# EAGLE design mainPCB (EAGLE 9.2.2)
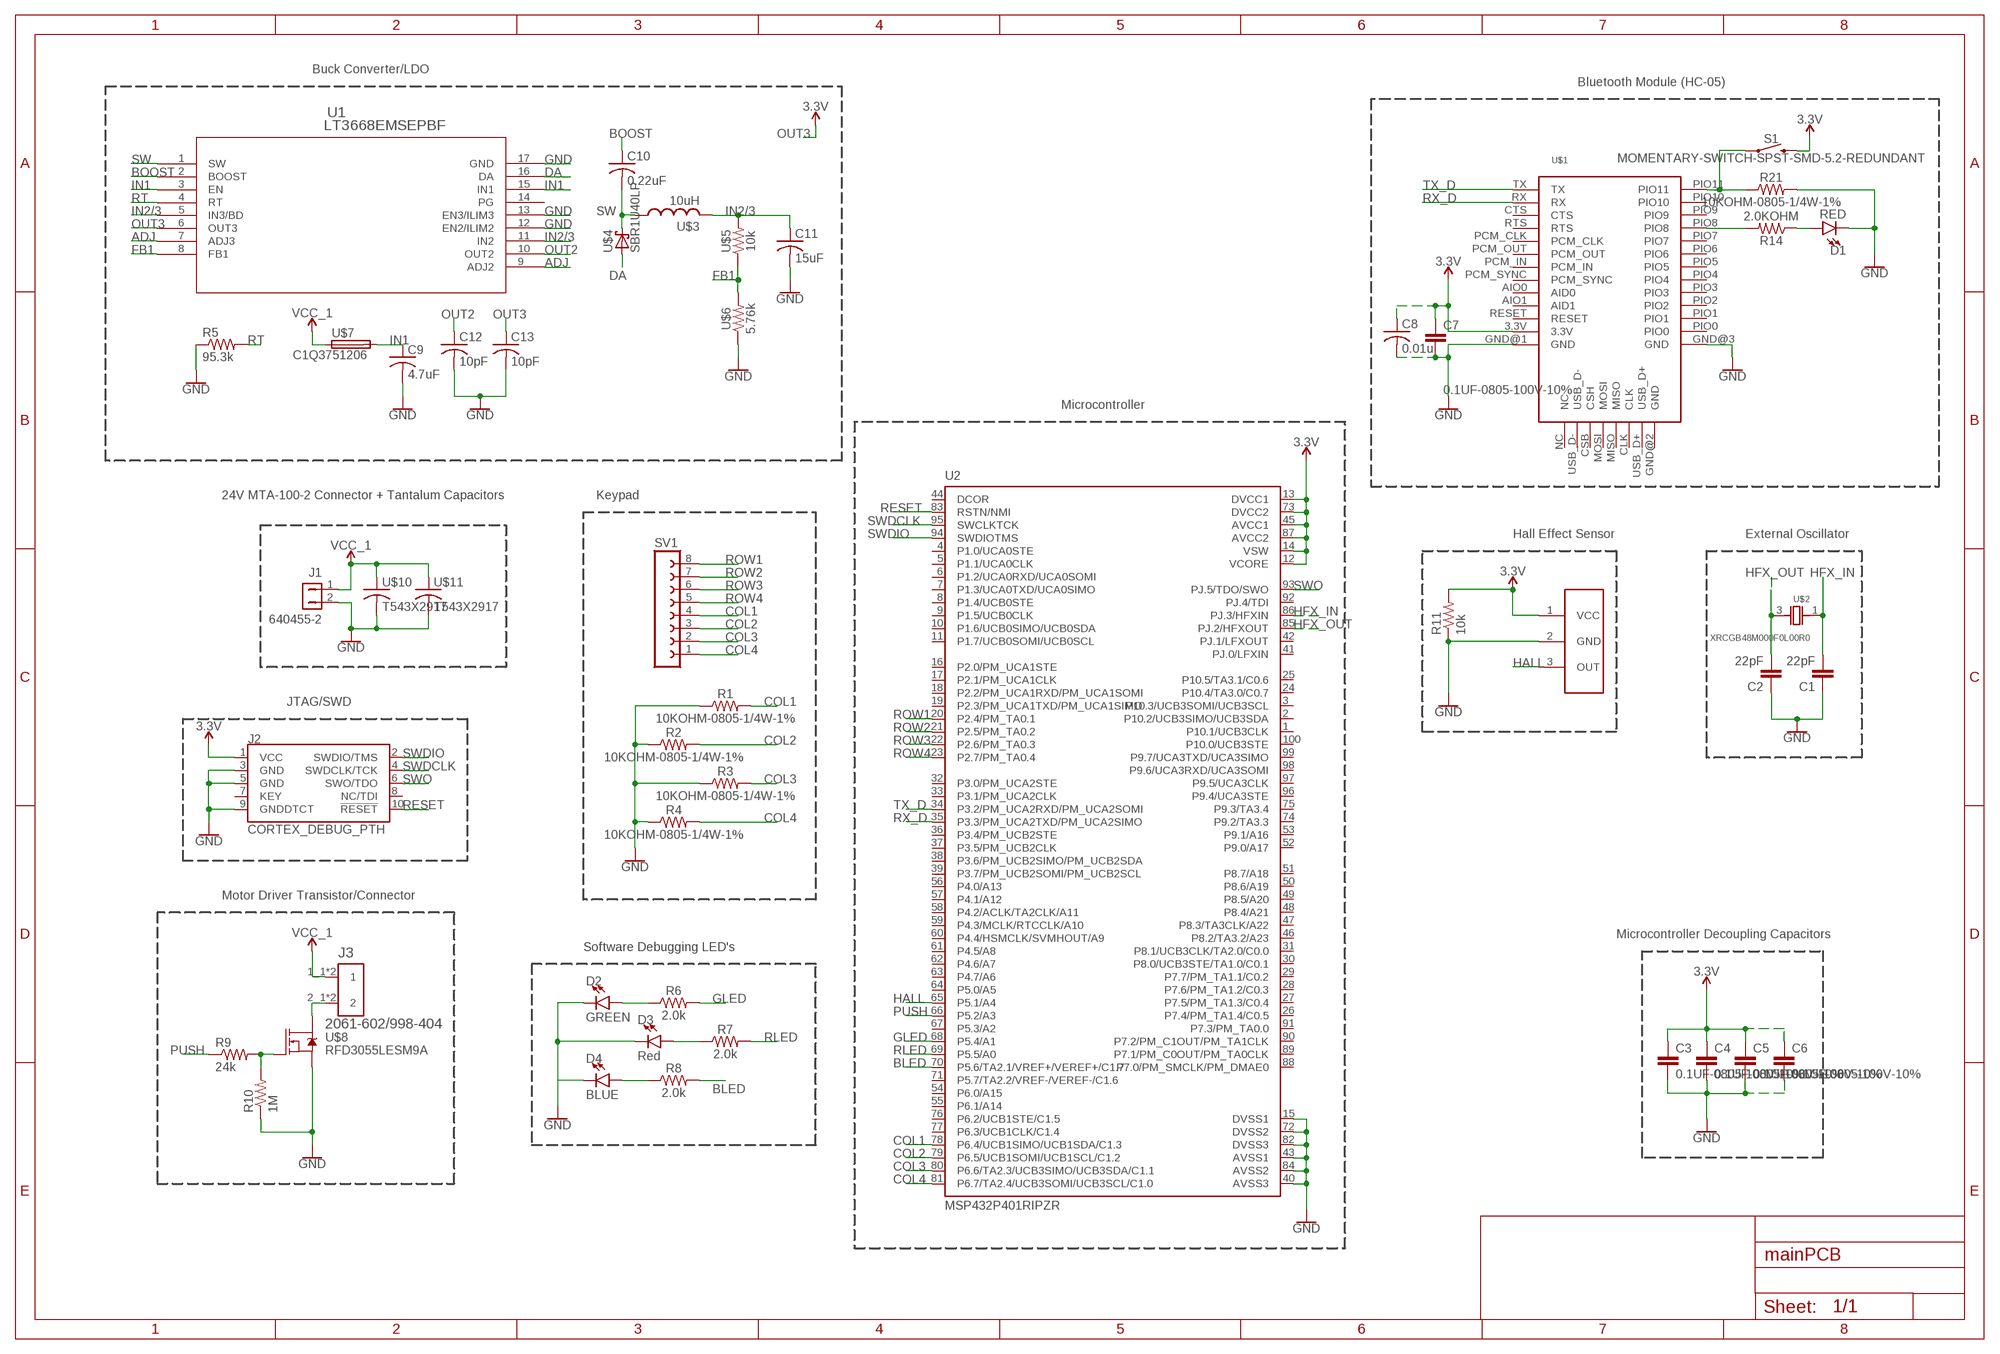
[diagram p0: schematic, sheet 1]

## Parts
C1  22pF  22PF-0603-50V-5%  [0603]
C2  22pF  22PF-0603-50V-5%  [0603]
C3  0.1UF-0805-100V-10%  [0805]
C4  0.1UF-0805-100V-10%  [0805]
C5  0.1UF-0805-100V-10%  [0805]
C6  0.1UF-0805-100V-10%  [0805]
C7  0.1UF-0805-100V-10%  [0805]
C8  0.01u  C-USC0805  [C0805]
C9  4.7uF  C-USC0805  [C0805]
C10  0.22uF  C-USC0805  [C0805]
C11  15uF  C-USC0805  [C0805]
C12  10pF  C-USC0805  [C0805]
C13  10pF  C-USC0805  [C0805]
D1  RED  LED-RED0603  [LED-0603]
D2  GREEN  LED-GREEN0603  [LED-0603]
D3  Red  LED-RED0603-SMART  [LED-0603]
D4  BLUE  LED-BLUE0603  [LED-0603]
J1  640455-2  [2-PIN_CONNECTOR]
J2  CORTEX_DEBUG_PTH  [2X5-PTH-1.27MM]
J3  2061-602/998-404  [WAGO_2061-602/998-404]
R1  10KOHM-0805-1/4W-1%  [0805]
R2  10KOHM-0805-1/4W-1%  [0805]
R3  10KOHM-0805-1/4W-1%  [0805]
R4  10KOHM-0805-1/4W-1%  [0805]
R5  95.3k  R-US_R0805  [R0805]
R6  2.0k  2.0KOHM-0603-1/10W-5%  [0603]
R7  2.0k  2.0KOHM-0603-1/10W-5%  [0603]
R8  2.0k  2.0KOHM-0603-1/10W-5%  [0603]
R9  24k  R-US_R0805  [R0805]
R10  1M  R-US_R0805  [R0805]
R11  10k  R-US_R0805  [R0805]
R14  2.0KOHM  [0805]
R21  10KOHM-0805-1/4W-1%  [0805]
S1  MOMENTARY-SWITCH-SPST-SMD-5.2-REDUNDANT  [TACTILE_SWITCH_SMD_5.2MM]
SV1  FE08-1  [FE08]
U1  LT3668EMSEPBF  [MSOP-16_MSE]
U2  MSP432P401RIPZR  [QFP50P1600X1600X160-100N]
U$1  HC-05  [HC-05_FOOTPRINT]
U$2  XRCGB48M000F0L00R0  [XTAL_XRCGB24M000F0L00R0]
U$3  10uH  CBC3225T150KR1210  [L3225M]
U$4  SBR1U40LP  [3-XDFN]
U$5  10k  ERJ-PB6  [R0805]
U$6  5.76k  ERJ-PB6  [R0805]
U$7  C1Q3751206  [C1206]
U$8  RFD3055LESM9A  [DPAK229P990X239-4N]
U$9  AH1807-P-B  [SIP3-UA]
U$10  T543X2917  [0204/5]
U$11  T543X2917  [0204/5]

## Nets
3.3V: C3.1 C4.1 C5.1 C6.1 C7.1 C8.1 J2.1(VCC) R11.2 S1.3 S1.4 U2.12(VCORE) U2.13(DVCC1) U2.14(VSW) U2.45(AVCC1) U2.73(DVCC2) U2.87(AVCC2) U$1.3.3V U$9.1(VCC)
ADJ: U1.7(ADJ3) U1.9(ADJ2)
BLED: R8.2 U2.70(P5.6/TA2.1/VREF+/VEREF+/C1.7)
BOOST: C10.1 U1.2(BOOST)
COL1: R1.2 SV1.4 U2.78(P6.4/UCB1SIMO/UCB1SDA/C1.3)
COL2: R2.2 SV1.3 U2.79(P6.5/UCB1SOMI/UCB1SCL/C1.2)
COL3: R3.2 SV1.2 U2.80(P6.6/TA2.3/UCB3SIMO/UCB3SDA/C1.1)
COL4: R4.2 SV1.1 U2.81(P6.7/TA2.4/UCB3SOMI/UCB3SCL/C1.0)
DA: U1.16(DA) U$4.1(A)
FB1: U1.8(FB1) U$5.1 U$6.2
GLED: R6.2 U2.68(P5.4/A1)
GND: C1.1 C2.1 C3.2 C4.2 C5.2 C6.2 C7.2 C8.2 C9.2 C11.2 C12.2 C13.2 D1.C D2.C D3.C J1.2 J2.3(GND) J2.5(GND) J2.9(GNDDTCT) R1.1 R2.1 R3.1 R4.1 R5.1 R10.1 R11.1 R21.2 U1.12(EN2/ILIM2) U1.13(EN3/ILIM3) U1.17(GND) U2.15(DVSS1) U2.40(AVSS3) U2.43(AVSS1) U2.72(DVSS2) U2.82(DVSS3) U2.84(AVSS2) U$1.GND@1(GND) U$1.GND@3(GND) U$6.1 U$8.3(S) U$9.2(GND) U$10.2 U$11.2
HALL: U2.65(P5.1/A4) U$9.3(OUT)
HFX_IN: C1.2 U2.86(PJ.3/HFXIN) U$2.1
HFX_OUT: C2.2 U2.85(PJ.2/HFXOUT) U$2.3
IN1: C9.1 U1.3(EN) U1.15(IN1) U$7.2
IN2/3: C11.1 U1.5(IN3/BD) U1.11(IN2) U$3.2 U$5.2
N$1: R9.2 R10.2 U$8.1(G)
N$2: J3.2_1 J3.2_2 U$8.4(D)
N$3: D1.A R14.1
N$4: D2.A R6.1
N$5: D3.A R7.1
N$8: D4.A R8.1
N$9: D4.C
N$11: R21.1 S1.1 S1.2 U$1.PIO11
N$19: R14.2 U$1.PIO8
OUT2: C12.1 U1.10(OUT2)
OUT3: C13.1 U1.6(OUT3) ; supply symbol labelled 3.3V
PUSH: R9.1 U2.66(P5.2/A3)
RESET: J2.10(!RESET) U2.83(RSTN/NMI)
RLED: R7.2 U2.69(P5.5/A0)
ROW1: SV1.8 U2.20(P2.4/PM_TA0.1)
ROW2: SV1.7 U2.21(P2.5/PM_TA0.2)
ROW3: SV1.6 U2.22(P2.6/PM_TA0.3)
ROW4: SV1.5 U2.23(P2.7/PM_TA0.4)
RT: R5.2 U1.4(RT)
RX_D: U2.35(P3.3/PM_UCA2TXD/PM_UCA2SIMO) U$1.RX
SW: C10.2 U1.1(SW) U$3.1 U$4.2(C) U$4.3(C)
SWDCLK: J2.4(SWDCLK/TCK) U2.95(SWCLKTCK)
SWDIO: J2.2(SWDIO/TMS) U2.94(SWDIOTMS)
SWO: J2.6(SWO/TDO) U2.93(PJ.5/TDO/SWO)
TX_D: U2.34(P3.2/PM_UCA2RXD/PM_UCA2SOMI) U$1.TX
VCC_1: J1.1 J3.1_1 J3.1_2 U$7.1 U$10.1 U$11.1
Unconnected: J2.7(KEY) J2.8(NC/TDI) U1.14(PG) U2.1(P10.1/UCB3CLK) U2.2(P10.2/UCB3SIMO/UCB3SDA) U2.3(P10.3/UCB3SOMI/UCB3SCL) U2.4(P1.0/UCA0STE) U2.5(P1.1/UCA0CLK) U2.6(P1.2/UCA0RXD/UCA0SOMI) U2.7(P1.3/UCA0TXD/UCA0SIMO) U2.8(P1.4/UCB0STE) U2.9(P1.5/UCB0CLK) U2.10(P1.6/UCB0SIMO/UCB0SDA) U2.11(P1.7/UCB0SOMI/UCB0SCL) U2.16(P2.0/PM_UCA1STE) U2.17(P2.1/PM_UCA1CLK) U2.18(P2.2/PM_UCA1RXD/PM_UCA1SOMI) U2.19(P2.3/PM_UCA1TXD/PM_UCA1SIMO) U2.24(P10.4/TA3.0/C0.7) U2.25(P10.5/TA3.1/C0.6) U2.26(P7.4/PM_TA1.4/C0.5) U2.27(P7.5/PM_TA1.3/C0.4) U2.28(P7.6/PM_TA1.2/C0.3) U2.29(P7.7/PM_TA1.1/C0.2) U2.30(P8.0/UCB3STE/TA1.0/C0.1) U2.31(P8.1/UCB3CLK/TA2.0/C0.0) U2.32(P3.0/PM_UCA2STE) U2.33(P3.1/PM_UCA2CLK) U2.36(P3.4/PM_UCB2STE) U2.37(P3.5/PM_UCB2CLK) U2.38(P3.6/PM_UCB2SIMO/PM_UCB2SDA) U2.39(P3.7/PM_UCB2SOMI/PM_UCB2SCL) U2.41(PJ.0/LFXIN) U2.42(PJ.1/LFXOUT) U2.44(DCOR) U2.46(P8.2/TA3.2/A23) U2.47(P8.3/TA3CLK/A22) U2.48(P8.4/A21) U2.49(P8.5/A20) U2.50(P8.6/A19) U2.51(P8.7/A18) U2.52(P9.0/A17) U2.53(P9.1/A16) U2.54(P6.0/A15) U2.55(P6.1/A14) U2.56(P4.0/A13) U2.57(P4.1/A12) U2.58(P4.2/ACLK/TA2CLK/A11) U2.59(P4.3/MCLK/RTCCLK/A10) U2.60(P4.4/HSMCLK/SVMHOUT/A9) U2.61(P4.5/A8) U2.62(P4.6/A7) U2.63(P4.7/A6) U2.64(P5.0/A5) U2.67(P5.3/A2) U2.71(P5.7/TA2.2/VREF-/VEREF-/C1.6) U2.74(P9.2/TA3.3) U2.75(P9.3/TA3.4) U2.76(P6.2/UCB1STE/C1.5) U2.77(P6.3/UCB1CLK/C1.4) U2.88(P7.0/PM_SMCLK/PM_DMAE0) U2.89(P7.1/PM_C0OUT/PM_TA0CLK) U2.90(P7.2/PM_C1OUT/PM_TA1CLK) U2.91(P7.3/PM_TA0.0) U2.92(PJ.4/TDI) U2.96(P9.4/UCA3STE) U2.97(P9.5/UCA3CLK) U2.98(P9.6/UCA3RXD/UCA3SOMI) U2.99(P9.7/UCA3TXD/UCA3SIMO) U2.100(P10.0/UCB3STE) U$1.AIO0(AID0) U$1.AIO1(AID1) U$1.CLK U$1.CSB(CSH) U$1.CTS U$1.GND@2(GND) U$1.MISO U$1.MOSI U$1.NC U$1.PCM_CLK U$1.PCM_IN U$1.PCM_OUT U$1.PCM_SYNC U$1.PIO0 U$1.PIO1 U$1.PIO2 U$1.PIO3 U$1.PIO4 U$1.PIO5 U$1.PIO6 U$1.PIO7 U$1.PIO9 U$1.PIO10 U$1.RESET U$1.RTS U$1.USB_D+ U$1.USB_D-

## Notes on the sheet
- Buck Converter/LDO
- Bluetooth Module (HC-05)
- Microcontroller
- 24V MTA-100-2 Connector + Tantalum Capacitors | Keypad
- Hall Effect Sensor | External Oscillator
- JTAG/SWD
- Motor Driver Transistor/Connector
- Microcontroller Decoupling Capacitors
- Software Debugging LED's

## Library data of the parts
C1 C2 = SparkFun-Capacitors:22PF: 22pF ceramic capacitors; PROD_ID: CAP-07876
C3-C7 = SENIOR_DESIGN_COMPONENTS:0.1UF: 0.1µF ceramic capacitors
C8-C13 = SENIOR_DESIGN_COMPONENTS:C-US: CAPACITOR, American symbol; SPICEPREFIX: C
D1 = SENIOR_DESIGN_COMPONENTS:LED-RED: Red SMD LED; PROD_ID: DIO-00819
D2 = SENIOR_DESIGN_COMPONENTS:LED-GREEN: Green SMD LED; PROD_ID: DIO-00821
D3 = SENIOR_DESIGN_COMPONENTS:LED-RED: Red SMD LED; PROD_ID: DIO-11154
D4 = SENIOR_DESIGN_COMPONENTS:LED-BLUE: Blue SMD LED; PROD_ID: DIO-08575
J1 = SENIOR_DESIGN_COMPONENTS:640455-2: 2 Pin Rectangular Connector; AVAILABILITY: Unavailable; COMMENT: 640455-2; DESCRIPTION: MTA-100 2 Position 2.54 mm Single Row Right Angle Wire to Board Header; EU_ROHS_COMPLIANCE: Compliant; MF: TE Connectivity; MP: 640455-2; PACKAGE: None; PRICE: None; TE_PURCHASE_URL: https://www.te.com/usa-en/product-640455-2.html?te_bu=Cor&te_type=disp&te_campaign=seda_glo_cor-seda-global-disp-prtnr-fy19-seda-model-bom-cta_sma-317_1&elqCampaignId=32493
J2 = SparkFun-Connectors:CORTEX_DEBUG: Cortex Debug Connector - 10 pin Supports JTAG debug, Serial Wire debug, and Serial Wire Viewer. PTH and SMD connector options available. General Connector Information Products: PTH Connector -via Digi-Key SparkFun PSoc SparkFun T
J3 = SENIOR_DESIGN_COMPONENTS:2061-602/998-404: 2061 Series 2 Position 20-16 AWG 6 mm Spacing Surface Mount Terminal Block; AVAILABILITY: Unavailable; DESCRIPTION: 2061 Series 2 Position 20-16 AWG 6 mm Spacing Surface Mount Terminal Block; MF: WAGO; MP: 2061-602/998-404; PACKAGE: None; PRICE: None
R1-R4 R21 = SENIOR_DESIGN_COMPONENTS:10KOHM: 10kΩ resistor
R5 R9-R11 = SENIOR_DESIGN_COMPONENTS:R-US_: RESISTOR, American symbol; SPICEPREFIX: R
R6-R8 = SENIOR_DESIGN_COMPONENTS:2.0KOHM: 2kΩ resistor; PROD_ID: RES-08296
R14 = SENIOR_DESIGN_COMPONENTS:2.0KOHM: 2kΩ resistor
S1 = SENIOR_DESIGN_COMPONENTS:MOMENTARY-SWITCH-SPST: Momentary Switch (Pushbutton) - SPST; PROD_ID: SWCH-08247; SF_SKU: COM-08720
SV1 = SENIOR_DESIGN_COMPONENTS:FE08-1: FEMALE HEADER; OC_FARNELL: unknown; OC_NEWARK: unknown
U1 = SENIOR_DESIGN_COMPONENTS:LT3668EMSEPBF; DESCRIPTION: LT3668 - 40V 400mA Step-Down Switching Regulator with Dual Fault Protected Tracking LDOs; DIGI-KEY_PART_NUMBER: LT3668EMSE#PBF-ND; DIGI-KEY_PURCHASE_URL: https://www.digikey.com/product-detail/en/linear-technology-analog-devices/LT3668EMSE-PBF/LT3668EMSE-PBF-ND/5030729?utm_source=snapeda&utm_medium=aggregator&utm_campaign=symbol; MF: Linear Technology; MP: LT3668EMSE#PBF; PACKAGE: MSOP-16 Linear Technology
U2 = SENIOR_DESIGN_COMPONENTS:MSP432P401RIPZR: Low-Power and High Performance 32-Bit ARM Cortex M4F With 256KB Flash and 64KB RAM 100-LQFP -40 to 85; AVAILABILITY: Unavailable; DESCRIPTION: Low-Power and High Performance 32-Bit ARM Cortex M4F With 256KB Flash and 64KB RAM 100-LQFP -40 to 85; MF: Texas Instruments; MP: MSP432P401RIPZR; PACKAGE: LQFP-100 Texas Instruments; PRICE: None
U$1 = SENIOR_DESIGN_COMPONENTS:HC-05
U$2 = SENIOR_DESIGN_COMPONENTS:XRCGB48M000F0L00R0
U$3 = SENIOR_DESIGN_COMPONENTS:CBC3225T150KR
U$4 = SENIOR_DESIGN_COMPONENTS:SBR1U40LP
U$5 U$6 = SENIOR_DESIGN_COMPONENTS:ERJ-PB6
U$7 = SENIOR_DESIGN_COMPONENTS:C1Q375
U$8 = SENIOR_DESIGN_COMPONENTS:RFD3055LESM9A
U$9 = SENIOR_DESIGN_COMPONENTS:AH1807-P-B
U$10 U$11 = SENIOR_DESIGN_COMPONENTS:T543X

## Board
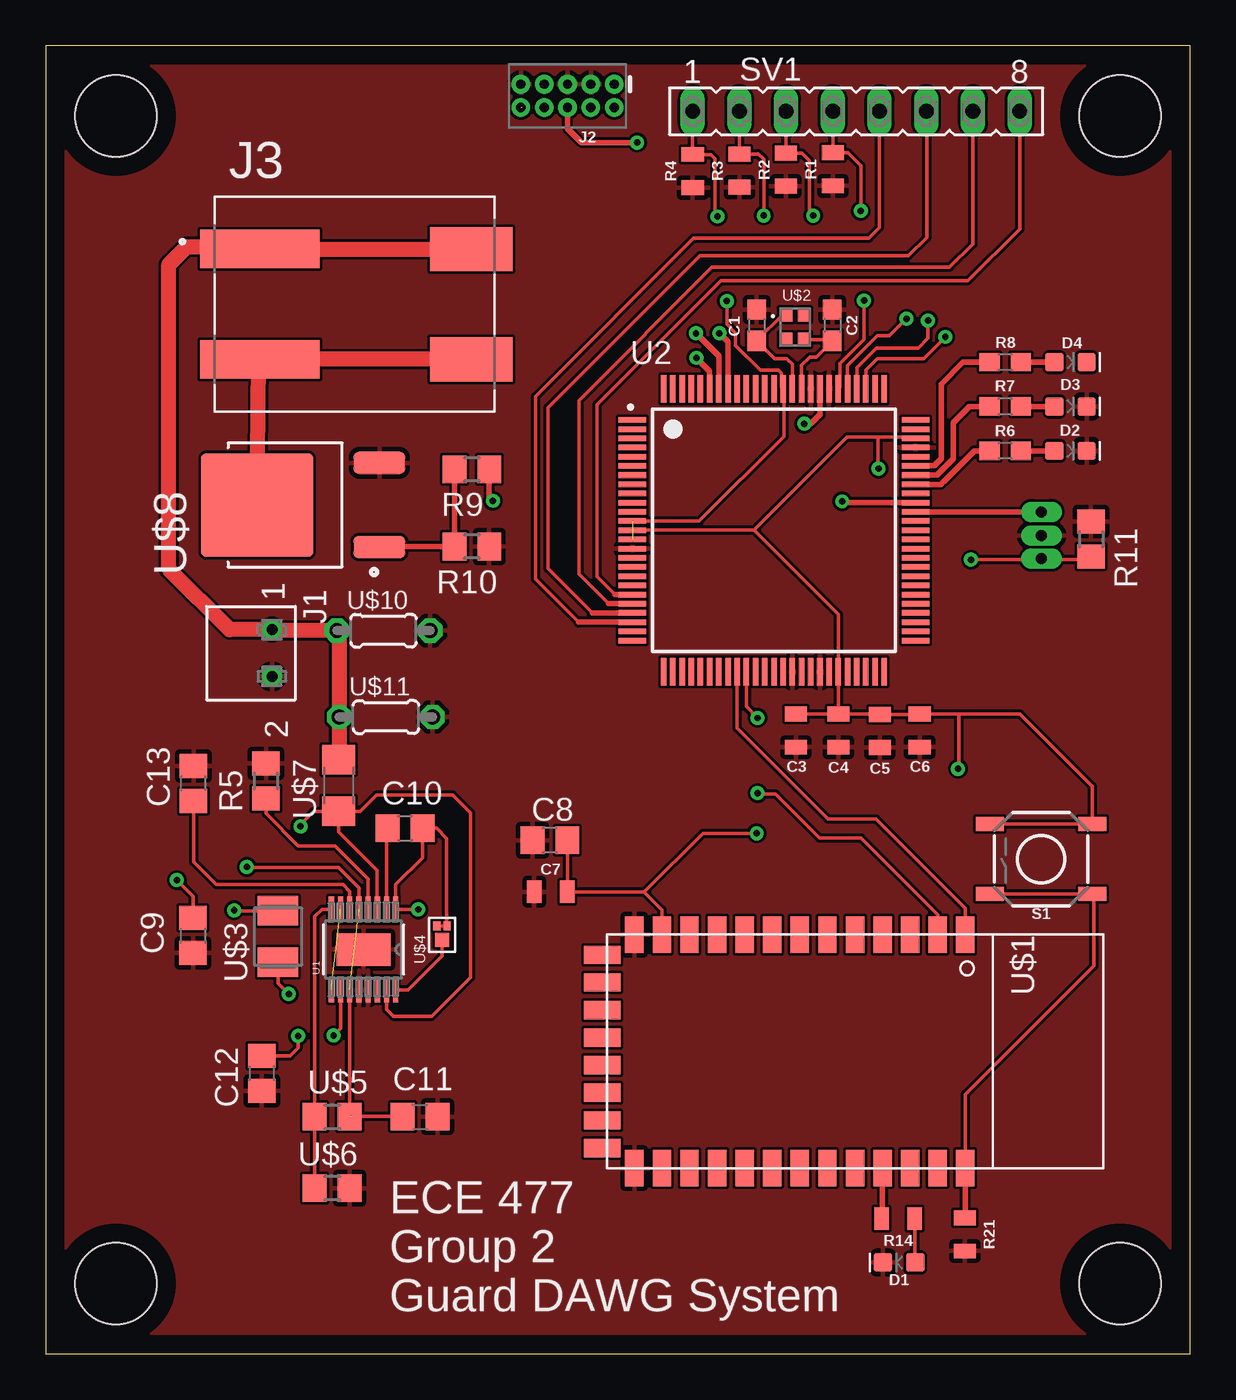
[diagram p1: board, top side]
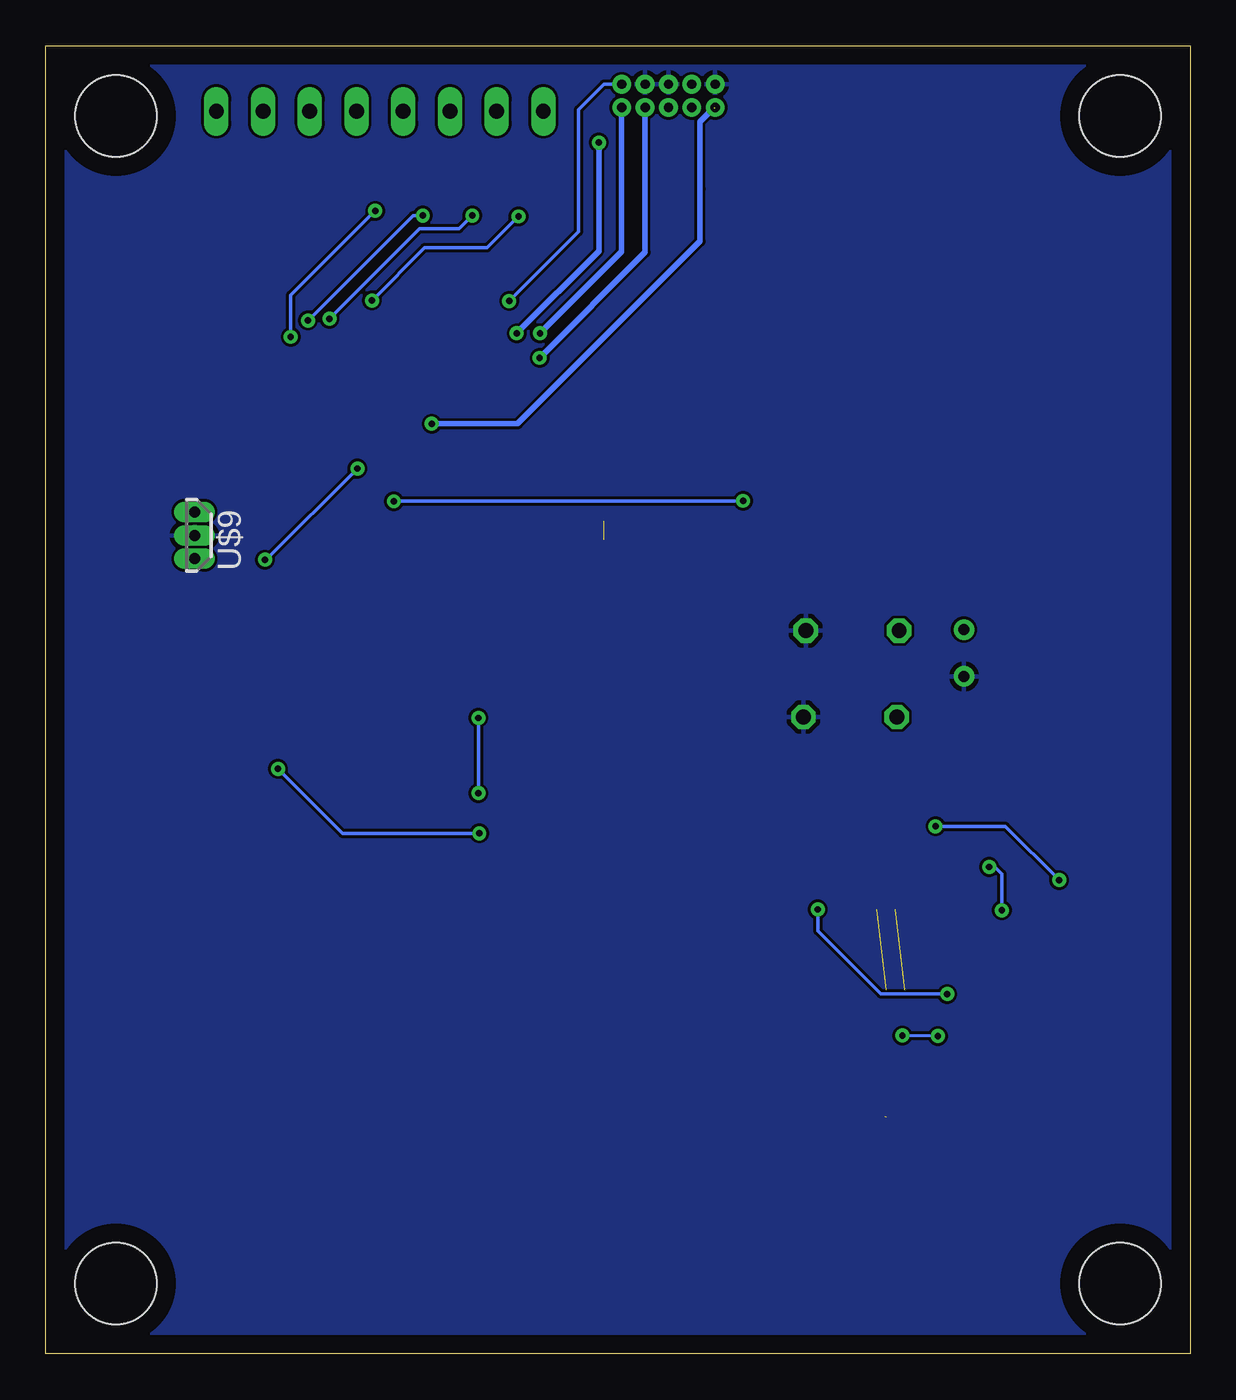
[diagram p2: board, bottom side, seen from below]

Size 62.23 x 71.12 mm. Coordinates in mm from the lower left corner, seen from the top.
Outline: 0,0 62.23,0 62.23,71.12 0,71.12 0,0
Copper layers (1*16): Top 0.035mm / dielectric 1.5mm / Bottom 0.035mm
Design rules "default": minimum track width 6mil, minimum drill 0.35mm, track to track 6mil, track to pad 6mil, pad to pad 6mil, via to via 6mil, smd to smd 6mil, copper to edge 40mil, drill to drill 6mil, minimum pad ring 10mil, minimum via ring 8mil, stop-mask expansion 4mil, vias tented up to drill 0mil, thermal gap 10mil
Holes 4.45 mm at 3.81,67.31 58.42,67.31 58.42,3.81 3.81,3.81

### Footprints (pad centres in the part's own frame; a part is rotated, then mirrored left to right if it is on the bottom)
0603 = smd 1.1 x 1: 1 -0.85,0; 2 0.85,0
0805 = smd 0.8 x 1.2: 1 -0.9,0; 2 0.9,0
C0805 = smd 1.3 x 1.5: 1 -0.95,0; 2 0.95,0
LED-0603 = smd 1 x 1: A -0.877,0; C 0.877,0
2-PIN_CONNECTOR = drill 0.6: 1 -1.27,0; 2 1.27,0
2X5-PTH-1.27MM = drill 0.508 pad 1: 1 -2.54,-0.635; 2 -2.54,0.635; 3 -1.27,-0.635; 4 -1.27,0.635; 5 0,-0.635; 6 0,0.635; 7 1.27,-0.635; 8 1.27,0.635; 9 2.54,-0.635; 10 2.54,0.635
WAGO_2061-602/998-404 = smd 6.5 x 2.1: 1_1 -5.15,3; 2_1 -5.15,-3 | smd 4.5 x 2.4: 1_2 6.35,3; 2_2 6.35,-3
R0805 = smd 1.3 x 1.5: 1 -0.95,0; 2 0.95,0
TACTILE_SWITCH_SMD_5.2MM = smd 1.524 x 0.762: 1 -2.794,1.905; 2 2.794,1.905; 3 -2.794,-1.905; 4 2.794,-1.905
FE08 = drill 0.813 long: 1 -8.89,0; 2 -6.35,0; 3 -3.81,0; 4 -1.27,0; 5 1.27,0; 6 3.81,0; 7 6.35,0; 8 8.89,0
MSOP-16_MSE = smd 1.397 x 0.279: 1 -2.184,1.751; 2 -2.184,1.251; 3 -2.184,0.751; 4 -2.184,0.25; 5 -2.184,-0.25; 6 -2.184,-0.751; 7 -2.184,-1.251; 8 -2.184,-1.751; 9 2.184,-1.751; 10 2.184,-1.251; 11 2.184,-0.751; 12 2.184,-0.25; 13 2.184,0.25; 14 2.184,0.751; 15 2.184,1.251; 16 2.184,1.751 | smd 1.753 x 2.946: 17 0,0
QFP50P1600X1600X160-100N = smd 1.5 x 0.3: 1 -7.7,6; 2 -7.7,5.5; 3 -7.7,5; 4 -7.7,4.5; 5 -7.7,4; 6 -7.7,3.5; 7 -7.7,3; 8 -7.7,2.5; 9 -7.7,2; 10 -7.7,1.5; 11 -7.7,1; 12 -7.7,0.5; 13 -7.7,0; 14 -7.7,-0.5; 15 -7.7,-1; 16 -7.7,-1.5; 17 -7.7,-2; 18 -7.7,-2.5; 19 -7.7,-3; 20 -7.7,-3.5; 21 -7.7,-4; 22 -7.7,-4.5; 23 -7.7,-5; 24 -7.7,-5.5; 25 -7.7,-6; 51 7.7,-6; 52 7.7,-5.5; 53 7.7,-5; 54 7.7,-4.5; 55 7.7,-4; 56 7.7,-3.5; 57 7.7,-3; 58 7.7,-2.5; 59 7.7,-2; 60 7.7,-1.5; 61 7.7,-1; 62 7.7,-0.5; 63 7.7,0; 64 7.7,0.5; 65 7.7,1; 66 7.7,1.5; 67 7.7,2; 68 7.7,2.5; 69 7.7,3; 70 7.7,3.5; 71 7.7,4; 72 7.7,4.5; 73 7.7,5; 74 7.7,5.5; 75 7.7,6 | smd 0.3 x 1.5: 26 -6,-7.7; 27 -5.5,-7.7; 28 -5,-7.7; 29 -4.5,-7.7; 30 -4,-7.7; 31 -3.5,-7.7; 32 -3,-7.7; 33 -2.5,-7.7; 34 -2,-7.7; 35 -1.5,-7.7; 36 -1,-7.7; 37 -0.5,-7.7; 38 0,-7.7; 39 0.5,-7.7; 40 1,-7.7; 41 1.5,-7.7; 42 2,-7.7; 43 2.5,-7.7; 44 3,-7.7; 45 3.5,-7.7; 46 4,-7.7; 47 4.5,-7.7; 48 5,-7.7; 49 5.5,-7.7; 50 6,-7.7; 76 6,7.7; 77 5.5,7.7; 78 5,7.7; 79 4.5,7.7; 80 4,7.7; 81 3.5,7.7; 82 3,7.7; 83 2.5,7.7; 84 2,7.7; 85 1.5,7.7; 86 1,7.7; 87 0.5,7.7; 88 0,7.7; 89 -0.5,7.7; 90 -1,7.7; 91 -1.5,7.7; 92 -2,7.7; 93 -2.5,7.7; 94 -3,7.7; 95 -3.5,7.7; 96 -4,7.7; 97 -4.5,7.7; 98 -5,7.7; 99 -5.5,7.7; 100 -6,7.7
HC-05_FOOTPRINT = smd 2 x 1: 3.3V 0,3; AIO0 0,7.5; AIO1 0,6; CTS 0,16.5; GND@1 0,1.5; GND@3 12.7,1.5; PCM_CLK 0,13.5; PCM_IN 0,10.5; PCM_OUT 0,12; PCM_SYNC 0,9; PIO0 12.7,3; PIO1 12.7,4.5; PIO2 12.7,6; PIO3 12.7,7.5; PIO4 12.7,9; PIO5 12.7,10.5; PIO6 12.7,12; PIO7 12.7,13.5; PIO8 12.7,15; PIO9 12.7,16.5; PIO10 12.7,18; PIO11 12.7,19.5; RESET 0,4.5; RTS 0,15; RX 0,18; TX 0,19.5 | smd 1 x 2: CLK 8.6,-0.25; CSB 4.1,-0.25; GND@2 11.6,-0.25; MISO 7.1,-0.25; MOSI 5.6,-0.25; NC 1.1,-0.25; USB_D+ 10.1,-0.25; USB_D- 2.6,-0.25
XTAL_XRCGB24M000F0L00R0 = smd 0.7 x 0.75: 1 -0.5,0.675; 2 -0.5,-0.675; 3 0.5,-0.675; 4 0.5,0.675
L3225M = smd 1.6 x 2.2: 1 -1.4,0; 2 1.4,0
3-XDFN = smd 0.75 x 0.75: 1 0,0 | smd 0.48 x 0.4: 2 0.76,0.275; 3 0.76,-0.275
C1206 = smd 1.6 x 1.8: 1 -1.4,0; 2 1.4,0
DPAK229P990X239-4N = smd 1.22 x 2.83: 1 -2.29,-4.14; 3 2.29,-4.14 | smd 5.63 x 6.1: 4 0,2.51
SIP3-UA = drill 0.6 pad 0.7 long: 1 -1.27,0; 2 0,0; 3 1.27,0
0204/5 = drill 0.813 octagon: 1 -2.54,0; 2 2.54,0

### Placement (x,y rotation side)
C1  38.66,55.93 270 top
C2  42.77,55.93 270 top
C3  40.79,33.88 270 top
C4  43.1,33.88 270 top
C5  45.36,33.86 270 top
C6  47.52,33.88 270 top
C7  27.46,25.12 180 top
C8  27.41,27.91 180 top
C9  8,22.73 270 top
C10  19.53,28.57 0 top
C11  20.35,12.88 0 top
C12  11.73,15.24 270 top
C13  8.03,31.01 90 top
D1  46.41,4.95 180 top
D2  55.73,49.1 0 top
D3  55.73,51.51 0 top
D4  55.73,53.92 0 top
J1  12.29,38.1 270 top
J2  28.37,68.4 180 top
J3  16.79,57.07 0 top
R1  42.8,64.41 90 top
R2  40.26,64.39 90 top
R3  37.72,64.34 90 top
R4  35.18,64.31 90 top
R5  11.96,31.14 270 top
R6  52.17,49.1 180 top
R7  52.17,51.51 180 top
R8  52.17,53.92 180 top
R9  23.16,48.08 180 top
R10  23.16,43.89 180 top
R11  56.85,44.3 270 top
R14  46.35,7.34 180 top
R21  49.99,6.48 270 top
S1  54.13,26.9 180 top
SV1  44.07,67.56 0 top
U1  17.27,21.97 270 top
U2  39.6,44.78 0 top
U$1  30.51,22.78 270 top
U$2  40.74,55.83 0 top
U$3  12.62,22.68 90 top
U$4  21.54,22.5 90 top
U$5  15.57,12.88 0 top
U$6  15.57,8.99 180 top
U$7  15.93,30.89 270 top
U$8  14,46.15 90 top
U$9  54.15,44.5 90 bottom
U$10  18.36,39.32 0 top
U$11  18.49,34.62 0 top

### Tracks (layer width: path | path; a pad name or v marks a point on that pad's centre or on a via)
3.3V  (via drill 0.35)  (2 unrouted)
  Top 0.2: S1.4 S1.3 56.92,30.84 52.97,34.78 49.66,34.78 | C3.1 C4.1 | C4.1 45.34,34.78 C5.1 47.5,34.76 C6.1 49.66,34.78 | U$1.3.3V 33.51,24.13 32.54,25.09 | 32.54,25.09 28.38,25.09 C7.1 C8.1 | R11.2 56.68,43.18 54.2,43.18 U$9.1 54.1,43.18 v50.32,43.18 | U2.12 35.53,45.28 40.13,49.89 40.13,52.45 U2.87 40,52.58 40,53.34 39.85,53.48 38.85,53.48 37.5,54.83 37.5,55.51 37.03,55.98 v37.03,57.25 | U2.13 38.51,44.78 | 38.51,44.78 43.56,49.84 45.26,49.84 | 45.26,49.84 47.24,49.84 U2.73 | 38.51,44.78 43.1,40.18 U2.45 C4.1 | 45.26,49.84 45.26,48.16 v45.29,48.13 | 32.54,25.09 35.74,28.3 v38.66,28.3 | v49.61,31.8 49.66,31.85 49.66,34.78
  Bottom 0.2: v45.29,48.13 50.24,43.18 v50.32,43.18 | v37.03,57.25 33.27,61.01 33.27,67.64 31.88,69.04 J2.1 | v38.66,28.3 46.1,28.3 v49.61,31.8
ADJ  (1 unrouted)
BLED
  Top 0.2: U2.70
  Top 0.305: R8.2 49.89,53.92 48.69,52.73 48.69,48.67 48.31,48.28 U2.70
BOOST
  Top 0.2: U1.2 18.52,28.52 C10.1
COL1  (via drill 0.35)
  Top 0.2: U2.78 44.6,53.49 45.24,54.13 47.75,54.13 v48.92,55.3 | v44.32,62.15 44.32,64.62 43.63,65.31 R1.2 SV1.4
  Bottom 0.2: v48.92,55.3 48.92,57.56 v44.32,62.15
COL2  (via drill 0.35)
  Top 0.2: U2.79 44.1,53.62 45.16,54.69 47.45,54.69 47.98,55.22 v47.98,56.19 | v41.73,61.9 41.53,62.1 41.53,64.87 41.11,65.29 R2.2 SV1.3
  Bottom 0.2: v47.98,56.19 42.27,61.9 v41.73,61.9
COL3  (via drill 0.35)
  Top 0.2: U2.80 43.6,53.73 45.23,55.36 45.89,55.36 v46.81,56.29 | v39.04,61.9 39.04,64.95 38.73,65.25 38.72,65.24 R3.2 SV1.2
  Bottom 0.2: v46.81,56.29 41.91,61.19 39.75,61.19 v39.04,61.9
COL4  (via drill 0.35)
  Top 0.2: U2.81 43.2,52.58 43.2,53.83 44.5,55.13 v44.5,57.28 | v36.52,61.85 36.4,61.98 36.4,65 36.18,65.21 R4.2 SV1.1
  Bottom 0.2: v44.5,57.28 41.63,60.15 38.23,60.15 v36.52,61.85
DA
  Top 0.2: U$4.1 21.54,21.61 19.71,19.79 U1.16
FB1
  Top 0.2: U1.8 15.01,24.16 14.62,23.76 U$5.1 U$6.2
GLED
  Top 0.2: 49.7,48.3 | 48.83,47.43 | 47.31,47.27 U2.68
  Top 0.305: R6.2 50.49,49.1 49.7,48.3 | 48.83,47.43 48.67,47.27 47.31,47.27 | 49.7,48.3 48.83,47.43
GND
  pour Top: 0,71.12 0,0 62.23,0.13 62.23,71.12
  pour Bottom: 0,71.12 0,0 62.23,0 62.23,71.12
HALL
  Top 0.2: U$9.3
  Top 0.305: U2.65 U$9.3
HFX_IN
  Top 0.2: U2.86 40.6,53.81 40.28,54.13 39.61,54.13 C1.2 40.08,56.5 U$2.1
HFX_OUT
  Top 0.2: U2.85 41.1,53.75 41.55,54.2 41.9,54.2 C2.2 42.7,55.15 U$2.3
IN1  (via drill 0.35)
  Top 0.2: U1.3 18.02,26.27 15.93,28.37 U$7.2 | C9.1 8,24.87 v7.11,25.76 | v13.84,28.68 13.84,28.78 14.55,29.49 U$7.2 | U$7.2 17.09,29.49 17.98,30.38 22.12,30.38 23.09,29.41 23.09,20.45 20.98,18.34 18.9,18.34 18.52,18.71 U1.15
  Bottom 0.2: v7.11,25.76 10.03,28.68 v13.84,28.68
IN2/3  (via drill 0.35)  (2 unrouted)
  Top 0.2: U$3.2 10.26,24.08 v10.24,24.11 | v10.92,26.47 10.95,26.44 15.91,26.44 17.02,25.33 U1.5 | C11.1 19.39,12.9 16.59,12.9 | U$5.2 U1.11
  Bottom 0.2: v10.24,24.11 10.24,26.09 10.62,26.47 v10.92,26.47
N$1
  Top 0.2: U$8.1 18.16,43.89
  Top 0.305: R9.2 R10.2 18.16,43.89
N$2
  Top 0.2: 11.56,53.99 J3.2_1
  Top 0.813: J3.2_2 J3.2_1 | U$8.4 11.56,53.99
N$3
  Top 0.2: R14.1 47.26,4.98 D1.A
N$4
  Top 0.305: R6.1 D2.A
N$5
  Top 0.305: R7.1 D3.A
N$8
  Top 0.305: R8.1 D4.A
N$11
  Top 0.2: S1.2 S1.1 57,24.92 57,21.08 50.01,14.09 U$1.PIO11 | R21.1 50.01,7.39
  Top 0.305: 50.01,7.39 U$1.PIO11
N$19
  Top 0.2: 45.51,7.39 R14.2
  Top 0.305: U$1.PIO8 45.51,7.39
OUT2  (via drill 0.35)
  Top 0.2: v15.65,17.3 16.02,17.67 U1.10 | v13.72,17.27 13.72,16.62 13.28,16.19 C12.1
  Bottom 0.2: v15.65,17.3 v13.72,17.27
OUT3
  Top 0.2: U1.6 16.52,25.14 16.15,25.5 9.27,25.5 8.03,26.75 C13.1
PUSH  (via drill 0.35)
  Top 0.305: U2.66 43.38,46.28 v43.31,46.35 | R9.1 24.11,46.57 v24.31,46.38
  Bottom 0.2: v43.31,46.35 24.33,46.35 v24.31,46.38 24.23,46.38
RESET  (via drill 0.35)  (1 unrouted)
  Top 0.305: U2.83 42.1,51.06 41.6,50.57 v41.25,50.57
  Bottom 0.305: v41.25,50.57 36.58,50.57 26.64,60.5 26.64,63.35 26.64,67 25.88,67.77
RLED
  Top 0.305: R7.2 50.22,51.51 49.35,50.64 49.35,48.67 48.46,47.78 U2.69
ROW1
  Top 0.2: 30.96,41.28 29.97,42.27 29.97,51.61 36.7,58.34 50.14,58.34 52.96,61.16 SV1.8
  Top 0.305: U2.20 30.96,41.28
ROW2
  Top 0.2: 30.59,40.78 28.98,42.39 28.98,51.84 36.22,59.08 49.15,59.08 50.42,60.35 SV1.7
  Top 0.305: U2.21 30.59,40.78
ROW3
  Top 0.2: 29.72,40.28 27.3,42.7 27.3,51.46 35.56,59.72 46.91,59.72 47.9,60.71 47.9,67.54 SV1.6
  Top 0.305: U2.22 29.72,40.28
ROW4
  Top 0.2: 28.98,39.78 26.62,42.14 26.62,52.05 35.23,60.66 44.76,60.66 45.34,61.24 SV1.5
  Top 0.305: U2.23 28.98,39.78
RT
  Top 0.2: U1.4 17.52,25.81 15.72,27.61 13.72,27.61 11.96,29.36 R5.2
RX_D  (via drill 0.35)
  Top 0.2: U$1.RX 48.51,23.86 44.32,28.04 42.06,28.04 39.67,30.43 38.76,30.43 v38.71,30.48 | v38.71,34.57 38.1,35.18 U2.35
  Bottom 0.2: v38.71,30.48 v38.71,34.57
SW  (via drill 0.35)
  Top 0.2: U1.1 19.02,25.5 20.48,26.96 C10.2 21.23,28.57 21.79,28.02 21.79,23.29 U$4.3 U$4.2 | U1.1 | U$3.1 12.62,20.14 v13.21,19.56 | v20.24,24.16 U1.1
  Bottom 0.2: v13.21,19.56 16.82,19.56 20.24,22.99 v20.24,24.16 20.24,24.18
SWDCLK  (via drill 0.35)
  Top 0.305: U2.95 36.1,53.44 v35.38,54.15
  Bottom 0.305: v35.38,54.15 29.64,59.89 J2.4
SWDIO  (via drill 0.35)
  Top 0.305: U2.94 36.6,54.26 v35.36,55.5
  Bottom 0.305: v35.36,55.5 30.91,59.94 J2.2
SWO  (via drill 0.35)
  Top 0.305: U2.93 37.1,55.03 v36.63,55.5 | v32.16,65.86 29.13,65.86 28.37,66.62 J2.6
  Bottom 0.305: v36.63,55.5 32.16,59.97 v32.16,65.86
TX_D
  Top 0.2: U2.34 37.6,34.03 42.55,29.08 45.14,29.08 50.01,24.21 U$1.TX
VCC_1
  Top 0.2: U$10.1 15.95,39.19 | 11.52,60.2 J3.1_1 | 15.95,32.31 U$7.1
  Top 0.813: J3.1_1 J3.1_2 | U$10.1 12.34,39.32 J1.1 9.98,39.37 6.68,42.67 6.68,59.23 7.64,60.2 11.52,60.2 | 15.95,39.19 U$11.1 15.95,32.31

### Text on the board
tPlace: ECE 477 / Group 2 / Guard DAWG System

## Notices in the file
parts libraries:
SparkFun-PowerSymbols: Licensing: Creative Commons ShareAlike 4.0 International - https://creativecommons.org/licenses/by-sa/4.0
